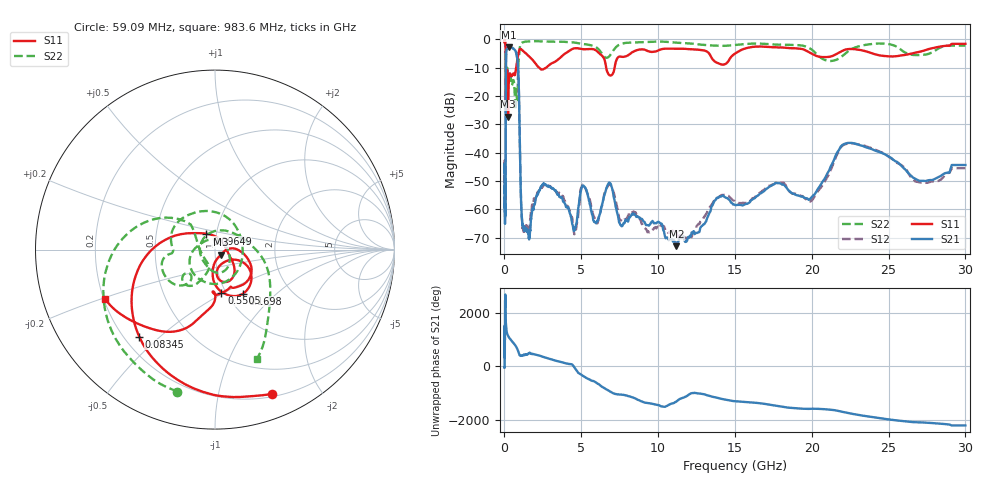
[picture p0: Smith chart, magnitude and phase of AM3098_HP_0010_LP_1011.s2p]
! Date/Time: Thu, Feb 28, 2019 8:33 AM
! Network Analyzer: Agilent Technologies E8364B Rev: A.07.50.67
! Sweep from 0.010 to 30.000 GHz, 1601 Points, Sweep Type: LOG
! Power Supply: 5.022 V, 0.002 A
# Hz S DB R 50
!freq MagS11 AngS11 MagS21 AngS21 MagS12 AngS12 MagS22 AngS22
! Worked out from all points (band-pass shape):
!   1601 points, 10 MHz to 30 GHz, reference 50 ohm
!   highest |S21| = -2.81 dB at 271.8 MHz (marker M1); lowest = -73.0 dB at 11.19 GHz (marker M2)
!   |S21| within 3 dB of the highest: 107.2 MHz to 807.2 MHz (699.9 MHz wide, 153 % of centre)
!   lowest |S11| = -27.3 dB at 233.9 MHz (marker M3), VSWR 1.09, Z = 53.3 - j2.95 ohm
!   |S11| at or under -10 dB: 92.12 MHz to 756.3 MHz (664.2 MHz wide, 157 % of centre); 2.272 GHz to 2.708 GHz (436.4 MHz wide, 17.5 % of centre); 6.622 GHz to 7.17 GHz (547.7 MHz wide, 7.94 % of centre)
!   |S22| runs from -24.9 to -0.6 dB; largest |S21 - S12| = 0.013
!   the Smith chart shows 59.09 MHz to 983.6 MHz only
!   S11 on the Smith chart (normalised r, x): 59.09 MHz: 0.23, -1.45; 83.45 MHz: 0.26, -0.43; 96.49 MHz: 0.89, +0.16; 169.8 MHz: 1.19, -0.64; 550.5 MHz: 0.95, -0.49; 983.6 MHz: 0.21, -0.21
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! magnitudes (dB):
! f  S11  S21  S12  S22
! 10 MHz  -0.4  -46.9  -43.3  -0.6
! 38.04 MHz  -0.5  -63.2  -59.9  -1.0
! 59.09 MHz  -1.3  -51.0  -52.5  -1.7
! 71.1 MHz  -1.9  -54.8  -57.3  -2.4
! 83.45 MHz  -3.8  -33.7  -33.3  -4.3
! 96.49 MHz  -19.9  -10.6  -10.6  -21.7
! 144.7 MHz  -15.0  -3.5  -3.5  -13.0
! 169.8 MHz  -10.7  -3.4  -3.4  -10.1
! 233.9 MHz  -27.3  -2.9  -2.9  -12.4
! 271.8 MHz  -16.4  -2.8  -2.8  -12.6
! 550.5 MHz  -12.2  -3.2  -3.1  -14.6
! 850.8 MHz  -6.6  -7.6  -7.6  -19.1
! 983.6 MHz  -3.5  -31.1  -31.0  -3.7
! 1.214 GHz  -4.1  -66.2  -66.8  -1.0
! 2.084 GHz  -8.9  -55.2  -55.4  -0.6
! 4.594 GHz  -3.1  -66.7  -67.9  -1.1
! 6.787 GHz  -12.4  -50.7  -51.3  -6.2
! 7.926 GHz  -5.9  -64.0  -63.5  -1.2
! 11.19 GHz  -3.3  -73.0  -68.1  -1.1
! 19.9 GHz  -4.7  -56.2  -57.3  -3.2
! 22.67 GHz  -3.4  -36.6  -36.7  -3.2
! 30 GHz  -1.6  -44.3  -45.5  -2.2
